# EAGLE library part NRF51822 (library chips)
Multiprotocol Bluetooth® 4.0 low energy/2.4 GHz RF SoC
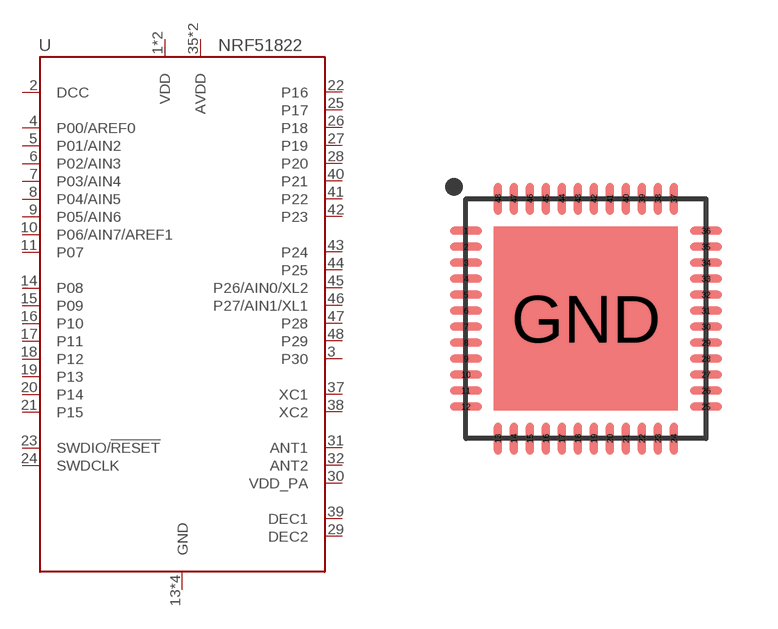
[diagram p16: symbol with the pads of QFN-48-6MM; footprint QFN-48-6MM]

Designator prefix U

## NRF51822QF (DIGIKEY: 1490-1049-1-ND; MANUFACTURER: Nordic Semi; MOUSER: 949-NRF51822-QFAC-R7; MPN: NRF51822-QFAC-R7)  [QFN-48-6MM]
1  VDD
2  DCC
3  P30
4  P00/AREF0
5  P01/AIN2
6  P02/AIN3
7  P03/AIN4
8  P04/AIN5
9  P05/AIN6
10  P06/AIN7/AREF1
11  P07
12  VDD
13  GND
14  P08
15  P09
16  P10
17  P11
18  P12
19  P13
20  P14
21  P15
22  P16
23  SWDIO/!RESET
24  SWDCLK
25  P17
26  P18
27  P19
28  P20
29  DEC2
30  VDD_PA
31  ANT1
32  ANT2
33  GND
34  GND
35  AVDD
36  AVDD
37  XC1
38  XC2
39  DEC1
40  P21
41  P22
42  P23
43  P24
44  P25
45  P26/AIN0/XL2
46  P27/AIN1/XL1
47  P28
48  P29
GND  GND

## Footprint QFN-48-6MM (pad centres in mm)
6MM x 6MM 48QFN package
smd 0.8 x 0.203: 1 -3,2.2; 2 -3,1.8; 3 -3,1.4; 4 -3,1; 5 -3,0.6; 6 -3,0.2; 7 -3,-0.2; 8 -3,-0.6; 9 -3,-1; 10 -3,-1.4; 11 -3,-1.8; 12 -3,-2.2; 25 3,-2.2; 26 3,-1.8; 27 3,-1.4; 28 3,-1; 29 3,-0.6; 30 3,-0.2; 31 3,0.2; 32 3,0.6; 33 3,1; 34 3,1.4; 35 3,1.8; 36 3,2.2
smd 0.203 x 0.8: 13 -2.2,-3; 14 -1.8,-3; 15 -1.4,-3; 16 -1,-3; 17 -0.6,-3; 18 -0.2,-3; 19 0.2,-3; 20 0.6,-3; 21 1,-3; 22 1.4,-3; 23 1.8,-3; 24 2.2,-3; 37 2.2,3; 38 1.8,3; 39 1.4,3; 40 1,3; 41 0.6,3; 42 0.2,3; 43 -0.2,3; 44 -0.6,3; 45 -1,3; 46 -1.4,3; 47 -1.8,3; 48 -2.2,3
smd 4.6 x 4.6: GND 0,0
